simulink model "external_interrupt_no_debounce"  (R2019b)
settings: Solver=FixedStepDiscrete  StartTime=0.0  StopTime=Inf  FixedStep=0.5  RelTol=1e-3  EnableMultiTasking=on
libraries: c2837xDlib x2, c2000lib x1, c280xlib x1

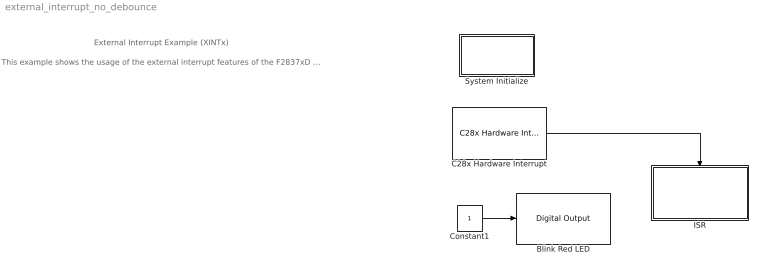
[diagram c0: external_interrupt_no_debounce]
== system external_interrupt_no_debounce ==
  note: This example shows the usage of the external interrupt features of the F2837xD board. These interrupts can be mapped to any GPIO on the board and utilized to enable an ISR. In this example pin 67 is mapped to XINT1 as a rising edge interrupt that toggles the blue LED each time it is triggered.. Requirements: 1. Enable the internal pull-up resistor on the pin of interest (they are disabled by default). EALLOW and EDIS are macros that enable and disable writing to the GPIO registers. 2. Set the interrupt to the correct XINTx CPU and PIE in the C28x Hardware Interrupt Block 3. Map the GPIO to XINTx under Model Settings -> Hardware Implementation -> Target hardware resources -> External Interrupt To do:
  note: External Interrupt Example (XINTx)
  Blink Red LED : c2837xDlib/Digital Output  GPIO_Number=GPIO32~GPIO39  GPIO_Bit0=off  GPIO_BIT0_Toggle=off  GPIO_Bit1=off  GPIO_BIT1_Toggle=off  GPIO_Bit2=on  GPIO_BIT2_Toggle=on  GPIO_Bit3=off  GPIO_BIT3_Toggle=off  GPIO_Bit4=off  GPIO_BIT4_Toggle=off  GPIO_Bit5=off  GPIO_BIT5_Toggle=off  GPIO_Bit6=off  GPIO_BIT6_Toggle=off  GPIO_Bit7=off  GPIO_BIT7_Toggle=on
  C28x Hardware Interrupt : c2000lib/Scheduling/C28x Hardware Interrupt  irqnumbers=1  pienumbers=4  irqpriorities=50  irqpreempts=1  showinput=off  dspchiptype=C280X
  Constant1 : Constant  OutDataTypeStr=boolean  SampleTime=1
  ISR : Subsystem
  System Initialize : Subsystem  mask(System Initialize){ShowInLibBrowser=0}
      mask prompts: ShowInLibBrowser "Simulink:masks:CustCodeMaskParam1_MP"
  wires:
  C28x Hardware Interrupt/1 -> ISR/Trigger
  Constant1/1 -> Blink Red LED/1

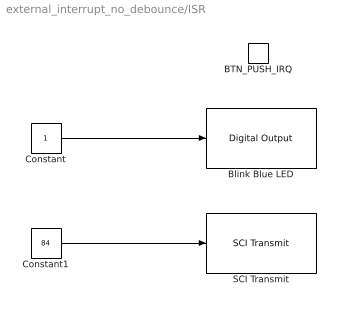
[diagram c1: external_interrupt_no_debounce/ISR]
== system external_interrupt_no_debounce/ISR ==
  BTN_PUSH_IRQ : TriggerPort  TriggerType=function-call  VariantControl=Variant  PortDimensions=1
  Blink Blue LED : c2837xDlib/Digital Output  GPIO_Number=GPIO24~GPIO31  GPIO_Bit0=off  GPIO_BIT0_Toggle=off  GPIO_Bit1=off  GPIO_BIT1_Toggle=off  GPIO_Bit2=off  GPIO_BIT2_Toggle=on  GPIO_Bit3=off  GPIO_BIT3_Toggle=off  GPIO_Bit4=off  GPIO_BIT4_Toggle=off  GPIO_Bit5=off  GPIO_BIT5_Toggle=off  GPIO_Bit6=off  GPIO_BIT6_Toggle=off  GPIO_Bit7=on  GPIO_BIT7_Toggle=on
  Constant : Constant
  Constant1 : Constant  Value=84  OutDataTypeStr=int16  SampleTime=-1
  SCI Transmit : c280xlib/SCI Transmit  sciModule=A  dataHead=''  dataTail=''  postInterrupt=off  numFifo=1
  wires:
  Constant/1 -> Blink Blue LED/1
  Constant1/1 -> SCI Transmit/1

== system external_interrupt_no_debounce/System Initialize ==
